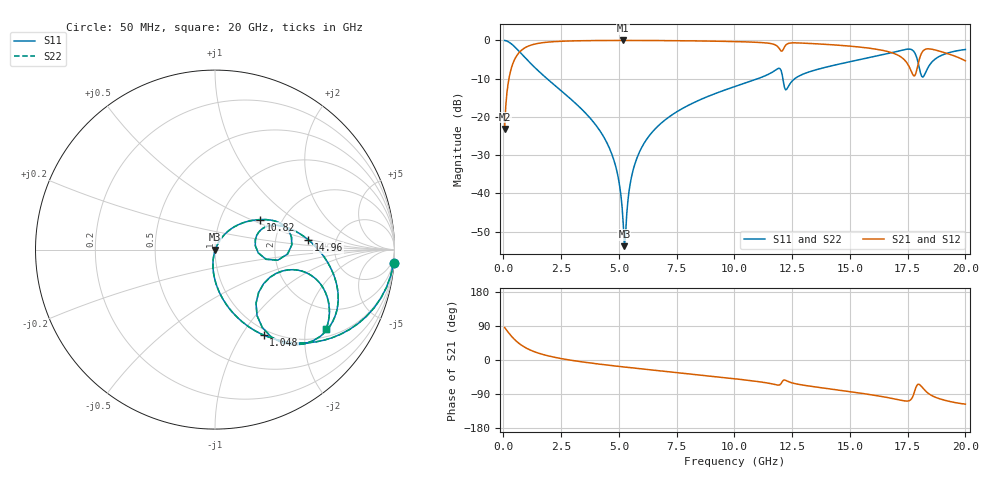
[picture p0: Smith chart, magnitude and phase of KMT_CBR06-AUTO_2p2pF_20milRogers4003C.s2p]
! Data measured by Modelithics Inc. support@modelithics.com 813-866-6335
! KEMET CBR06-AUTO 2.2pF, Pad Width= 0.851mm, Pad Length= 0.64mm, Pad Gap= 0.62mm, 20mil Rogers 4003C substrate Data, January 2022
# hz S ma R 50
! 2 Port Network Data from SP1.SP block
! freq  magS11  angS11  magS21  angS21  magS12  angS12  magS22  angS22
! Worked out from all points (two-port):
!   401 points, 50 MHz to 20 GHz, reference 50 ohm
!   highest |S21| = -0.02 dB at 5.187 GHz (marker M1); lowest = -23.1 dB at 50 MHz (marker M2)
!   |S21| within 3 dB of the highest: 702.8 MHz to 16.7 GHz (16 GHz wide, 184 % of centre); 18.14 GHz to 18.99 GHz (858.1 MHz wide, 4.62 % of centre)
!   lowest |S11| = -53.8 dB at 5.237 GHz (marker M3), VSWR 1.00, Z = 50.2 - j0.124 ohm
!   |S11| at or under -10 dB: 1.884 GHz to 11.01 GHz (9.13 GHz wide, 142 % of centre); 12.1 GHz to 12.62 GHz (517.9 MHz wide, 4.19 % of centre)
!   |S22| runs from -53.8 to 0.0 dB; largest |S21 - S12| = 0
!   S11 on the Smith chart (normalised r, x): 50 MHz: 1, -27; 1.048 GHz: 0.92, -1.26; 10.82 GHz: 1.54, +0.57; 14.96 GHz: 3.12, +0.46; 20 GHz: 1.25, -2.60
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5e7  0.9975 -4.2  0.06982 85.8  0.06982 85.8  0.9975 -4.2
3.99125e8  0.8715 -30.7  0.4894 59.2  0.4894 59.2  0.8715 -30.7
1.0475e9  0.5485 -60.3  0.8348 29.5  0.8348 29.5  0.5485 -60.3
3.391625e9  0.1258 -94.0  0.9902 -4.8  0.9902 -4.8  0.1258 -94.0
4.688375e9  0.03286 -101.5  0.9974 -14.8  0.9974 -14.8  0.03286 -101.5
4.987625e9  0.01505 -99.5  0.9978 -16.8  0.9978 -16.8  0.01505 -99.5
5.187125e9  0.003971 -79.0  0.9979 -18.2  0.9979 -18.2  0.003971 -79.0
5.237e9  0.002047 -37.0  0.9979 -18.5  0.9979 -18.5  0.002047 -37.0
5.73575e9  0.02671 63.9  0.9974 -21.8  0.9974 -21.8  0.02671 63.9
6.73325e9  0.07809 60.2  0.9946 -28.3  0.9946 -28.3  0.07809 60.2
1.0025e10  0.2499 39.6  0.9646 -49.6  0.9646 -49.6  0.2499 39.6
1.0823e10  0.3016 33.7  0.948 -55.4  0.948 -55.4  0.3016 33.7
1.206988e10  0.3544 -9.6  0.7257 -57.2  0.7257 -57.2  0.3544 -9.6
1.226938e10  0.2316 13.8  0.8929 -55.2  0.8929 -55.2  0.2316 13.8
1.336662e10  0.3991 19.0  0.9084 -69.9  0.9084 -69.9  0.3991 19.0
1.496262e10  0.5233 5.9  0.8431 -83.2  0.8431 -83.2  0.5233 5.9
1.670825e10  0.679 -12.4  0.7057 -100.0  0.7057 -100.0  0.679 -12.4
1.74065e10  0.7613 -27.5  0.5368 -108.3  0.5368 -108.3  0.7613 -27.5
1.775562e10  0.7242 -46.5  0.3456 -91.4  0.3456 -91.4  0.7242 -46.5
1.805488e10  0.3766 -52.6  0.6301 -66.9  0.6301 -66.9  0.3766 -52.6
1.845388e10  0.4785 -13.9  0.7742 -90.6  0.7742 -90.6  0.4785 -13.9
2e10  0.7598 -35.4  0.5407 -116.4  0.5407 -116.4  0.7598 -35.4
